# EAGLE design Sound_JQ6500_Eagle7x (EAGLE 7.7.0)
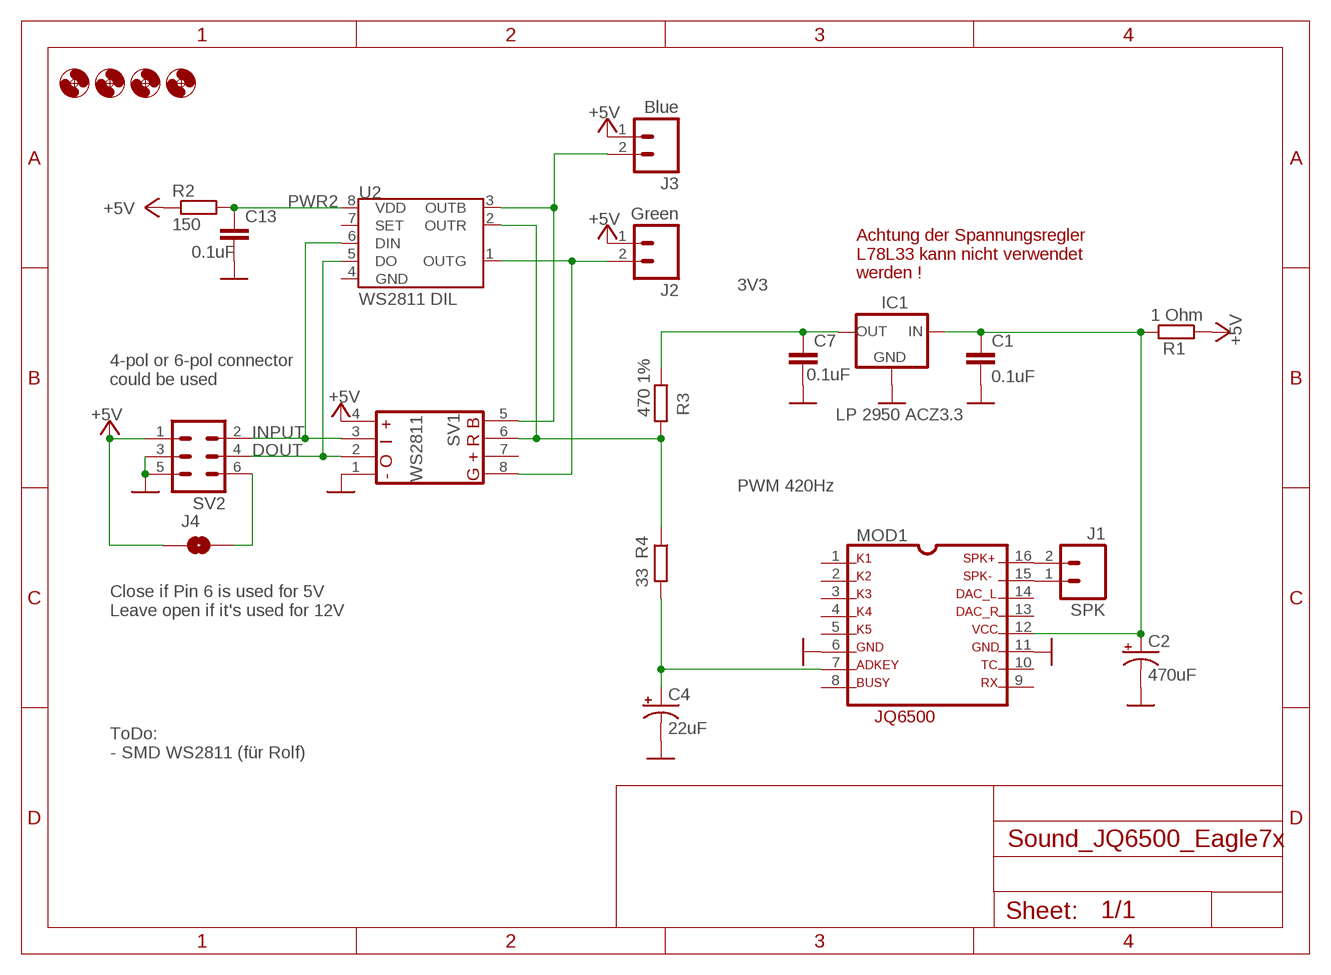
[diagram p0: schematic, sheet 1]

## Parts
C1  0.1uF  0.1UF-50V-20%(PTH)KIT-EZ  [CAP-PTH-SMALL-KIT]
C2  470uF  SPARKFUN-CAPACITORS_100UF-25V-20%(PTH)  [SPARKFUN-CAPACITORS_CPOL-RADIAL-100UF-25V]
C4  22uF  CAPACITORS_22UF  [CAPACITOR_CPOL-RADIAL-22UF]
C7  0.1uF  0.1UF-50V-20%(PTH)KIT-EZ  [CAP-PTH-SMALL-KIT]
C13  0.1uF  0.1UF-50V-20%(PTH)KIT-EZ  [CAP-PTH-SMALL-KIT]
H1  MOUNT-HOLE3.0  [3,0]
H2  MOUNT-HOLE3.0  [3,0]
H3  MOUNT-HOLE3.0  [3,0]
H4  MOUNT-HOLE3.0  [3,0]
IC1  LP 2950 ACZ3.3  78LXX  [78LXX]
J1  SPK  M02PTH  [1X02]
J2  Green  M02PTH  [1X02]
J3  Blue  M02PTH  [1X02]
J4  SOLDERJUMPERNO  [SJ_2S-NO]
MOD1  JQ6500  [JQ6500]
R1  1 Ohm  RCL_R-EU_0204/5  [RCL_0204/5]
R2  150  RCL_R-EU_0204/5  [RCL_0204/5]
R3  470 1%  RCL_R-EU_0204/5  [RCL_0204/5]
R4  33  RCL_R-EU_0204/5  [RCL_0204/5]
SV1  S3PO_MODUL_WS2811_SOUND_MP3-TF-16P_WS2811_AND_ATTINY_PUSHBUTTONACTION_4017_2_WS28115V  [S3PO_MODUL_WS2811_SOUND_MP3-TF-16P_WS2811_AND_ATTINY_PUSHBUTTONACTION_4017_2_WS2811_WS2811_5V]
SV2  ML6  [ML6]
U2  WS2811 DIL  S3PO_MODUL_WS2811_SOUND_MP3-TF-16P_WS2811_AND_ATTINY_WS2811-ICTINY45-20-DIP  [S3PO_MODUL_WS2811_SOUND_MP3-TF-16P_WS2811_AND_ATTINY_WS2811_DIP08]

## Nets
3V3: C7.1 IC1.OUT R3.1
+5V: J2.1 J3.1 J4.1 R1.1 R2.1 SV1.4(GND) SV2.1
B2: J3.2 SV1.5(OUTG) U2.3(OUTB)
DOUT: SV1.2(DIN) SV2.4 U2.5(DO)
G2: J2.2 SV1.8(OUTB) U2.1(OUTG)
GND: C1.2 C2.2(-) C4.2(-) C7.2 C13.2 IC1.GND MOD1.6 MOD1.11 SV1.1(VDD) SV2.3 SV2.5
INPUT: SV1.3(DO) SV2.2 U2.6(DIN)
N$1: J1.1 MOD1.15
N$2: J1.2 MOD1.16
N$3: C1.1 C2.1(+) IC1.IN MOD1.12 R1.2
N$4: J4.2 SV2.6
N$7: C4.1(+) MOD1.7 R4.2
PWR2: C13.1 R2.2 U2.8(VDD)
R1: R3.2 R4.1 SV1.6(OUT+) U2.2(OUTR)
Unconnected: MOD1.1 MOD1.2 MOD1.3 MOD1.4 MOD1.5 MOD1.8 MOD1.9 MOD1.10 MOD1.13 MOD1.14 SV1.7(OUTR) U2.7(SET)

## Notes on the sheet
- Achtung der Spannungsregler
  L78L33 kann nicht verwendet
  werden !
- 4-pol or 6-pol connector
  could be used
- PWM 420Hz
- Close if Pin 6 is used for 5V
  Leave open if it's used for 12V
- ToDo:
  - SMD WS2811 (für Rolf)

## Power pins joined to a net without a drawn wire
GND: U2.4(GND)

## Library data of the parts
C1 C7 C13 = SparkFun-Capacitors:0.1UF-50V-20%(PTH): CAP-08370; PROD_ID: CAP-08370
C2 = Sound_MP3-TF-16P_and_WS2811:SPARKFUN-CAPACITORS_100UF-25V-20%(PTH): CAP-08439; PROD_ID: CAP-08439
C4 = Sound_MP3-TF-16P_WS2811_and_ATTiny:CAPACITORS_22UF: CAP-08439; PROD_ID: CAP-08439
H1-H4 = holes:MOUNT-HOLE: MOUNTING HOLE with drill center marker
IC1 = v-reg-3:78LXX: VOLTAGE REGULATOR
J1-J3 = SparkFun-Connectors:M02: Standard 2-pin 0.1" header. Use with
J4 = SparkFun-Retired:SOLDERJUMPER: Solder Jumper
MOD1 = Sound_JQ6500:JQ6500: MP3-TF-16P http://www.electronicoscaldas.com/datasheet/DFR0299-DFPlayer-Mini-Manual.pdf; OC_FARNELL: unknown; OC_NEWARK: unknown
R1-R4 = Sound_MP3-TF-16P_and_WS2811:RCL_R-EU_: RESISTOR, European symbol; SPICEPREFIX: R
SV1 = S3PO_Modul_WS2811:S3PO_MODUL_WS2811_SOUND_MP3-TF-16P_WS2811_AND_ATTINY_PUSHBUTTONACTION_4017_2_WS2811: Modified by Hardi
SV2 = con-harting-ml:ML6: HARTING; OC_FARNELL: unknown; OC_NEWARK: unknown
U2 = S3PO_Modul_WS2811:S3PO_MODUL_WS2811_SOUND_MP3-TF-16P_WS2811_AND_ATTINY_WS2811-IC: Die Pin nummern im Dokument https://cdn-shop.adafruit.com/datasheets/WS2811.pdf für R und G sind vertauscht ;-(; PROD_ID: IC-09439; VALUE: TINY45-20-DIP

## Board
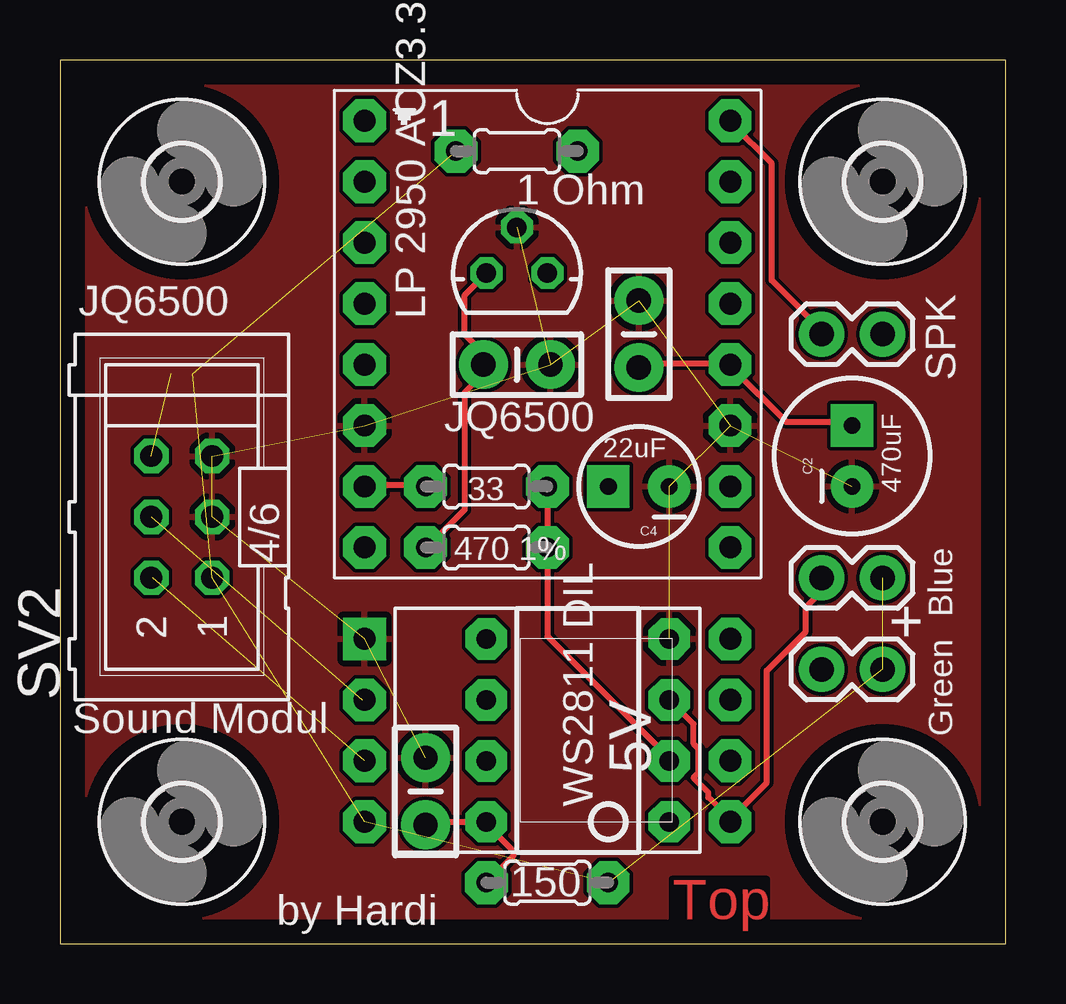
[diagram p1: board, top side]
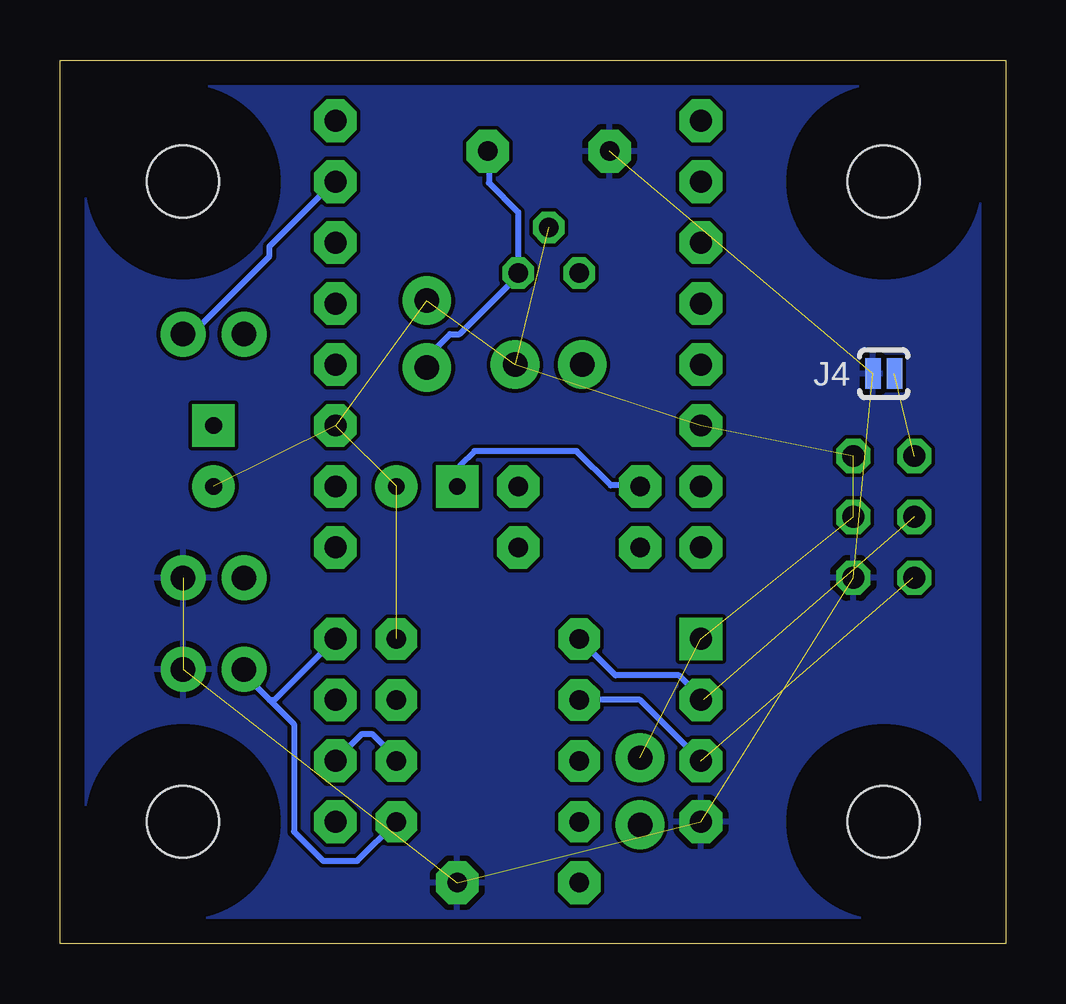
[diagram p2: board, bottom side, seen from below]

Size 39.42 x 36.82 mm. Coordinates in mm from the lower left corner, seen from the top.
Outline: 0,0 39.42,0 39.42,36.82 0,36.82 0,0
Copper layers (1*16): Top 0.035mm / dielectric 1.5mm / Bottom 0.035mm
Design rules "default *": minimum track width 10mil, minimum drill 0.35mm, track to track 6mil, track to pad 6mil, pad to pad 6mil, via to via 6mil, smd to smd 6mil, copper to edge 40mil, drill to drill 6mil, minimum pad ring 10mil, minimum via ring 8mil, stop-mask expansion 4mil, vias tented up to drill 0mil, thermal gap 10mil

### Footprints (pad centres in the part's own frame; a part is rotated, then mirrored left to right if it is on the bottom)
CAP-PTH-SMALL-KIT = drill 1.016 pad 2.032: 1 -1.397,0; 2 1.397,0
SPARKFUN-CAPACITORS_CPOL-RADIAL-100UF-25V = drill 0.7 pad 1.778 square: 1 1.27,0 | drill 0.7 pad 1.778: 2 -1.27,0
CAPACITOR_CPOL-RADIAL-22UF = drill 0.7 pad 1.778 square: 1 1.27,0 | drill 0.7 pad 1.778: 2 -1.27,0
3,0 = hole 3: 0,0
78LXX = drill 0.813 octagon: GND 0,1.905; IN 1.27,0; OUT -1.27,0
1X02 = drill 1.016 pad 1.88: 1 0,0; 2 2.54,0
SJ_2S-NO = smd 0.635 x 1.27: 1 -0.45,0; 2 0.45,0
JQ6500 = drill 0.914 pad 1.778 octagon: 1 -8.89,16.51; 2 -8.89,13.97; 3 -8.89,11.43; 4 -8.89,8.89; 5 -8.89,6.35; 6 -8.89,3.81; 7 -8.89,1.27; 8 -8.89,-1.27; 9 6.35,-1.27; 10 6.35,1.27; 11 6.35,3.81; 12 6.35,6.35; 13 6.35,8.89; 14 6.35,11.43; 15 6.35,13.97; 16 6.35,16.51
RCL_0204/5 = drill 0.813 pad 1.778 octagon: 1 -2.54,0; 2 2.54,0
S3PO_MODUL_WS2811_SOUND_MP3-TF-16P_WS2811_AND_ATTINY_PUSHBUTTONACTION_4017_2_WS2811_WS2811_5V = drill 0.914 pad 1.778 square: 1 -5.08,-5.08 | drill 0.914 pad 1.778 octagon: 2 -2.54,-5.08; 3 0,-5.08; 4 2.54,-5.08; 5 2.54,10.16; 6 0,10.16; 7 -2.54,10.16; 8 -5.08,10.16
ML6 = drill 0.914 octagon: 1 -2.54,-1.27; 2 -2.54,1.27; 3 0,-1.27; 4 0,1.27; 5 2.54,-1.27; 6 2.54,1.27
S3PO_MODUL_WS2811_SOUND_MP3-TF-16P_WS2811_AND_ATTINY_WS2811_DIP08 = drill 0.813 pad 1.727 octagon: 1 -3.81,-3.81; 2 -1.27,-3.81; 3 1.27,-3.81; 4 3.81,-3.81; 5 3.81,3.81; 6 1.27,3.81; 7 -1.27,3.81; 8 -3.81,3.81

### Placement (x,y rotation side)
C1  24.13,25.4 90 top
C2  33.02,20.32 90 top
C4  24.13,19.05 180 top
C7  19.05,24.13 0 top
C13  15.24,6.35 90 top
H1  34.29,5.08 0 top
H2  5.08,31.75 0 top
H3  5.08,5.08 0 top
H4  34.29,31.75 0 top
IC1  19.05,27.94 0 top
J1  34.29,25.4 180 top
J2  34.29,11.43 180 top
J3  34.29,15.24 180 top
J4  5.08,23.75 0 bottom
MOD1  21.59,17.78 0 top
R1  19.05,33.02 0 top
R2  20.32,2.54 180 top
R3  17.78,16.51 0 top
R4  17.78,19.05 180 top
SV1  17.78,7.62 270 top
SV2  5.08,17.78 90 top
U2  21.59,8.89 90 top

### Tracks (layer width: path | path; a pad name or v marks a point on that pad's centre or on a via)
3V3
  Top 0.254: IC1.OUT 16.87,27.03 16.87,25.4 17.48,24.79 17.48,24.18 C7.1 17.48,23.98 17.48,23.57 16.87,22.96 16.87,18.09 15.85,17.07 15.65,17.07 15.24,16.66 R3.1
+5V  (6 unrouted)
  pour Bottom: 0,0 39.37,0 39.37,36.83 0,36.83
B2
  Top 0.254: U2.3 26.42,9.14 26.42,8.33 26.62,8.13 26.62,7.11 26.42,6.91 27.03,6.3 27.03,6.1 28.04,5.08 SV1.5 27.84,5.08 29.46,6.71 29.46,11.38 31.09,13.01 31.09,14.02 31.7,14.63 31.7,15.24 J3.2
DOUT  (1 unrouted)
  Bottom 0.254: U2.5 16.26,11.18 13.61,11.18 12.6,10.16 SV1.2
G2
  Bottom 0.254: U2.1 27.03,3.45 28.45,3.45 29.67,4.67 29.67,9.14 30.68,10.16 | 30.68,10.16 31.9,11.38 J2.2 | SV1.8 30.48,10.16 30.68,10.16
GND  (11 unrouted)
  pour Top: 0,0 39.37,0 39.37,36.83 0,36.83
INPUT  (1 unrouted)
  Top 0.254: 3.86,15.24 SV2.2 | 12.6,7.52 SV1.3
  Bottom 0.254: U2.6 15.24,10.16 SV1.3
N$1
  Bottom 0.254: J1.1 33.93,25.4 30.68,28.65 30.68,29.06 28.04,31.7 MOD1.15
N$2
  Top 0.254: MOD1.16 28.04,34.14 29.67,32.51 29.67,27.64 31.9,25.4 J1.2
N$3
  Top 0.254: C1.1 24.18,24.18 27.84,24.18 MOD1.12 28.04,23.98 30.28,21.74 32.92,21.74 C2.1
  Bottom 0.254: R1.2 21.54,32.92 21.54,31.7 20.32,30.48 IC1.IN 20.32,27.84 22.76,25.4 23.16,25.4 23.98,24.59 23.98,24.18 C1.1
N$4  (1 unrouted)
N$7
  Top 0.254: MOD1.7 12.8,19.1 15.24,19.1 R4.2
  Bottom 0.254: C4.1 22.76,19.1 22.76,19.91 22.15,20.52 17.88,20.52 16.46,19.1 15.24,19.1 R4.2
PWR2
  Top 0.254: 17.68,5.08 15.24,5.08 C13.1 | R2.2 18.9,3.66 18.9,3.86 17.68,5.08 | 17.68,5.08 U2.8
R1
  Top 0.254: R4.1 R3.2 20.32,12.8 25.4,7.72 U2.2
  Bottom 0.254: SV1.6 26.82,8.74 26.42,8.74 25.4,7.72 U2.2

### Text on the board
Top: Top
tNames: JQ6500 | 4/ | + | Sound Modul | by Hardi

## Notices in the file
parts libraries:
SparkFun-Capacitors: Licensing: Creative Commons ShareAlike 4.0 International - https://creativecommons.org/licenses/by-sa/4.0
